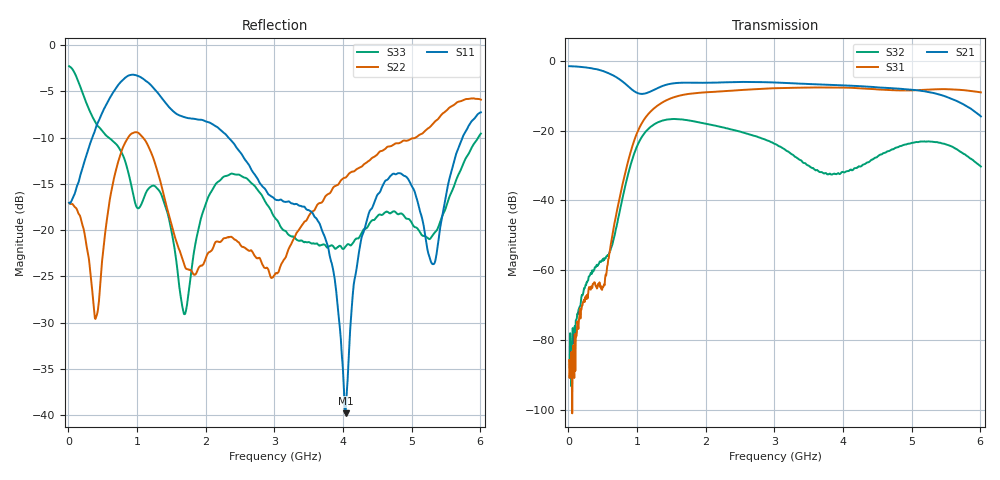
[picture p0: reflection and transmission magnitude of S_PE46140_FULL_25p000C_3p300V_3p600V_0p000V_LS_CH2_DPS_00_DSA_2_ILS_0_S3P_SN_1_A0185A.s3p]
! Device ID: PE46140_FULL
! File Path: z:\PE46140\MajorStates\25p000C\3p300\LS_CH2_DPS_00_DSA_2_ILS_0\PE46140_FULL_25p000C_3p300V_3p600V_0p000V_LS_CH2_DPS_00_DSA_2_ILS_0_S3P_SN_1_A0185A.s3p
! Serial: 1
! Lot: A0185A
! Temp: 25.000C
! VDD: 3.300
! VSS: 0.000
! Control_Hi: 3.600
! Control_Lo: 0.000
! Logic State: LS_CH2_DPS_00_DSA_2_ILS_0
! Port 1: RFIN
! Port 2: RFOUT1
! Port 3: RFOUT2
! ThroughPath:1-3
! IDD: 0.0003147783
! ISS: -1.071e-007
! Comment:
#  Hz  S  RI  R  50
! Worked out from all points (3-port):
!   801 points, 10 MHz to 6.01 GHz, reference 50 ohm
!   strongest paths, dB at 10 MHz, 1.51 GHz, 3.01 GHz, 4.51 GHz, 6.01 GHz:
!     S21: -1.5, -6.5, -6.2, -7.6, -15.9
!     S31: -85.8, -10.6, -7.8, -8.2, -9.0
!     S32: -87.0, -16.7, -23.8, -27.3, -30.3
!   lowest |S11| = -39.8 dB at 4.037 GHz (marker M1), VSWR 1.02, Z = 49 + j0.289 ohm
!   |S11| at or under -10 dB: start of sweep to 346.1 MHz; 2.331 GHz to 5.742 GHz (3.411 GHz wide, 84.5 % of centre)
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1e7  0.1402 -0.0109  0.8419 -0.0245  -1.91e-05 -7.81e-06
     0.8418 -0.0244  0.14 -0.00678  -3.17e-05 3.97e-05
     1.95e-05 4.74e-05  4.22e-05 -1.51e-05  0.766 -0.0725
3.55e8  -0.016 -0.3218  0.4591 -0.6282  -0.000524 -0.000258
        0.4592 -0.6262  -0.00907 -0.0427  -0.000105 0.00098
        -0.000552 -0.000314  -8.77e-05 0.000943  -0.361 -0.1865
1.165e9  -0.5852 0.2233  -0.2051 -0.2878  -0.1718 -0.0252
         -0.2053 -0.2886  0.2133 -0.1869  -0.00235 0.1064
         -0.1721 -0.0255  -0.00261 0.1064  0.1398 0.0917
1.69e9  -0.2866 0.2904  -0.4882 -0.0128  0.2272 0.2382
        -0.4884 -0.0129  0.0339 -0.0552  -0.0125 -0.1427
        0.2274 0.2386  -0.0124 -0.1426  -0.0338 -0.00959
3.01e9  0.0251 0.1444  0.4082 0.2724  -0.351 -0.2044
        0.408 0.2733  -0.0577 -0.00148  0.0577 -0.0283
        -0.3514 -0.2047  0.0576 -0.0286  0.1136 -0.0252
3.7525e9  0.0207 0.0853  0.2862 -0.3558  -0.2283 0.3492
          0.2868 -0.3558  0.0754 0.1338  -0.0157 0.019
          -0.2279 0.3494  -0.0157 0.0191  0.0819 0.000672
4.0375e9  -0.00981 0.00295  0.0426 -0.4424  -0.00661 0.4143
          0.0431 -0.4426  0.1393 0.1325  0.0214 0.0143
          -0.00545 0.4142  0.0216 0.0142  0.0816 -0.000762
4.4875e9  -0.1335 -0.0719  -0.3172 -0.2746  0.2921 0.2617
          -0.317 -0.2754  0.2413 0.0785  -0.0037 -0.0411
          0.2925 0.2613  -0.00387 -0.0413  0.1149 -0.0232
5.32e9  -0.0432 -0.0493  -0.1201 0.3254  0.2947 -0.2575
        -0.1207 0.3253  0.3779 -0.0347  0.00697 0.0686
        0.295 -0.2571  0.00705 0.0689  0.0941 0.0137
6.01e9  -0.3066 -0.306  0.153 0.0476  -0.1739 -0.3075
        0.1532 0.048  0.2471 -0.443  0.0262 -0.0158
        -0.1752 -0.3081  0.0261 -0.016  0.3107 0.1185
